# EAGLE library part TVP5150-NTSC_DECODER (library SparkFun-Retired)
Texas Instrument NTSC/PAL Decoder TI Part #TVP5150AM1 *** UNPROVEN FOOTPRINT *** Decodes NTSC video signal to YCbCr 4:2:2 signal Retired: IC-09311 Retired: IC-09080
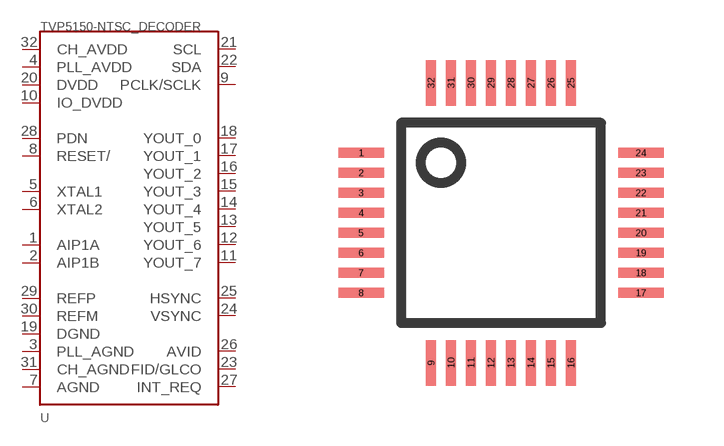
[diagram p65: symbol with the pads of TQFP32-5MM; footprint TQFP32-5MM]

Designator prefix -

## TVP5150-NTSC_DECODER  [TQFP32-5MM]
1  AIP1A
2  AIP1B
3  PLL_AGND
4  PLL_AVDD
5  XTAL1
6  XTAL2
7  AGND
8  RESET/
9  PCLK/SCLK
10  IO_DVDD
11  YOUT_7
12  YOUT_6
13  YOUT_5
14  YOUT_4
15  YOUT_3
16  YOUT_2
17  YOUT_1
18  YOUT_0
19  DGND
20  DVDD
21  SCL
22  SDA
23  FID/GLCO
24  VSYNC
25  HSYNC
26  AVID
27  INT_REQ
28  PDN
29  REFP
30  REFM
31  CH_AGND
32  CH_AVDD

## Footprint TQFP32-5MM (pad centres in mm)
smd 1.143 x 0.254: 1 -3.5,1.75; 2 -3.5,1.25; 3 -3.5,0.75; 4 -3.5,0.25; 5 -3.5,-0.25; 6 -3.5,-0.75; 7 -3.5,-1.25; 8 -3.5,-1.75; 17 3.5,-1.75; 18 3.5,-1.25; 19 3.5,-0.75; 20 3.5,-0.25; 21 3.5,0.25; 22 3.5,0.75; 23 3.5,1.25; 24 3.5,1.75
smd 0.254 x 1.143: 9 -1.75,-3.5; 10 -1.25,-3.5; 11 -0.75,-3.5; 12 -0.25,-3.5; 13 0.25,-3.5; 14 0.75,-3.5; 15 1.25,-3.5; 16 1.75,-3.5; 25 1.75,3.5; 26 1.25,3.5; 27 0.75,3.5; 28 0.25,3.5; 29 -0.25,3.5; 30 -0.75,3.5; 31 -1.25,3.5; 32 -1.75,3.5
